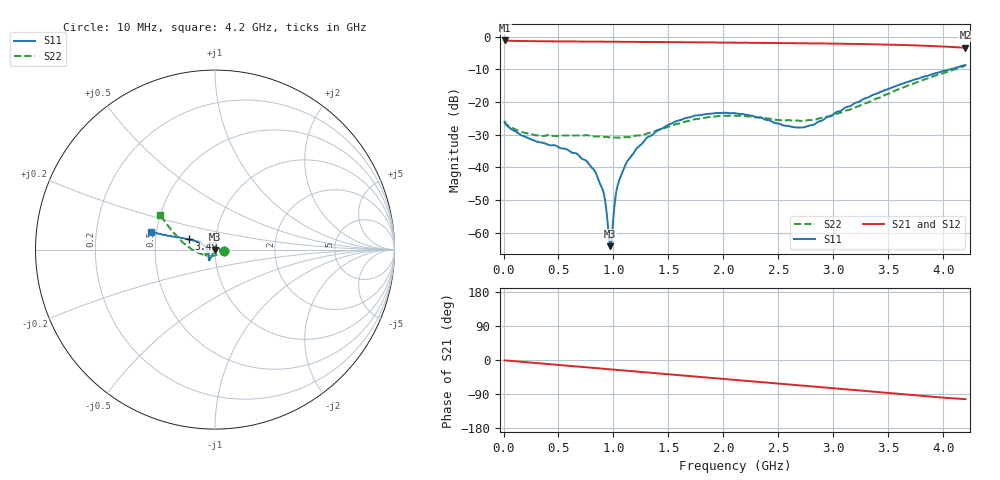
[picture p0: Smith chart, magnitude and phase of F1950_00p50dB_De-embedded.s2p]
! Integrated Device Technology
! Corporate Headquarters
! 6024 Silver Creek Valley Road
! San Jose, CA 95138  USA
! Phone:  1-408-284-8200
! Toll Free:  1-800-223-1366
! Webpage:  http://www.idt.com/
! Timing and RF Division
! 515 Groton Road, Suite 102
! Westford, MA 01886-6024
! Device:  F1950
! Description: 7-bit 0.25 dB Digital Step Attenuator
! Frequency:  150.0 -  4000.00 MHz
! Package:  4x4 mm Thin QFN Plastic Package: 24 pin
! Ports:  2 RF, 12 DC
!  Pin  1  = D0
!  Pin  2  = VDD
!  Pin  3  = Vmode
!  Pin  4  = GND
!  Pin  5  = RF1  =  Port 1
!  Pin  6  = GND
!  Pin  7  = GND
!  Pin  8  = GND
!  Pin  9  = GND
!  Pin 10  = GND
!  Pin 11  = GND
!  Pin 12  = GND
!  Pin 13  = GND
!  Pin 14  = RF2  =  Port 2
!  Pin 15  = GND
!  Pin 16  = LE
!  Pin 17  = CLK
!  Pin 18  = DATE
!  Pin 19  = D6
!  Pin 20  = D5
!  Pin 21  = D4
!  Pin 22  = D3
!  Pin 23  = D2
!  Pin 24  = D1
! State:  2
! Atten State:  0.50 dB
! Voltage:  +5.00 Volts
! Current:  Not Measured mA
! Data:  The device was measured on a the F195X evaluation board which has
!  individual transmission lines to the RF pins.  Data was collected
!  using a calibrated network analyzer.  The evaluation board was
!  de-embedded using a TRL calibration technique.
!  The reference plane is the edge of the package pin.
! Misc:  Board 2019
!  Action Tracker AT0250
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# GHz S dB R 50
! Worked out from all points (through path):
!   420 points, 10 MHz to 4.2 GHz, reference 50 ohm
!   highest |S21| = -1.10 dB at 10 MHz (marker M1); lowest = -3.3 dB at 4.2 GHz (marker M2)
!   group delay of S21, straight-line fit = 68.5 ps
!   lowest |S11| = -64.1 dB at 970 MHz (marker M3), VSWR 1.00, Z = 50.1 - j0.011 ohm
!   |S11| at or under -10 dB: start of sweep to 4.055 GHz
!   |S22| runs from -30.9 to -8.9 dB; largest |S21 - S12| = 0.0011
!   S11 on the Smith chart (normalised r, x): 10 MHz: 1.10, -0.02; 3.49 GHz: 0.74, +0.09; 4.2 GHz: 0.47, +0.11
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0.01  -26.09 -11.1  -1.10 -1.1  -1.10 -1.1  -25.78 -11.7
0.12  -29.22 -8.8  -1.25 -3.7  -1.25 -3.7  -28.60 -9.2
0.29  -31.94 9.6  -1.33 -8.0  -1.33 -8.0  -30.12 -5.0
0.57  -34.38 36.9  -1.41 -14.8  -1.41 -14.8  -30.21 -3.4
0.71  -37.26 45.5  -1.43 -18.2  -1.43 -18.2  -30.24 -12.3
0.82  -40.61 47.8  -1.45 -20.8  -1.45 -20.9  -30.51 -20.6
0.89  -45.89 52.5  -1.47 -22.5  -1.47 -22.6  -30.57 -28.4
0.92  -49.34 54.6  -1.48 -23.3  -1.47 -23.3  -30.63 -31.7
0.96  -61.73 24.5  -1.48 -24.2  -1.48 -24.3  -30.77 -37.5
0.97  -64.14 -10.2  -1.49 -24.5  -1.49 -24.5  -30.85 -38.9
0.99  -59.60 -92.7  -1.49 -25.0  -1.49 -25.0  -30.87 -41.2
1.03  -46.71 -117.2  -1.50 -25.9  -1.50 -26.0  -30.84 -48.3
1.1  -39.91 -120.6  -1.52 -27.6  -1.51 -27.6  -30.73 -59.4
1.22  -33.87 -117.8  -1.54 -30.5  -1.54 -30.6  -30.23 -79.4
1.41  -28.53 -117.1  -1.58 -35.2  -1.58 -35.2  -28.53 -108.5
1.74  -24.15 -117.3  -1.67 -43.2  -1.67 -43.3  -25.23 -138.1
2.11  -23.39 -120.3  -1.78 -52.3  -1.77 -52.3  -24.19 -153.0
2.64  -27.69 -158.2  -1.93 -65.3  -1.92 -65.3  -25.70 -152.0
2.81  -27.04 176.4  -1.99 -69.5  -1.98 -69.6  -25.54 -150.5
3.49  -16.09 158.4  -2.37 -87.0  -2.36 -87.0  -17.56 178.6
3.51  -15.82 158.7  -2.38 -87.5  -2.38 -87.5  -17.33 177.5
4.2  -8.64 164.2  -3.35 -103.2  -3.34 -103.3  -8.89 147.7
